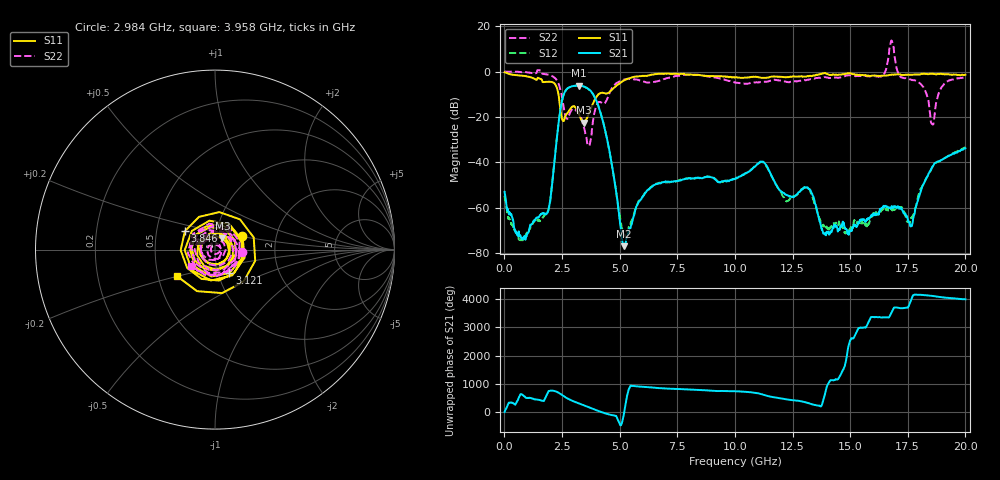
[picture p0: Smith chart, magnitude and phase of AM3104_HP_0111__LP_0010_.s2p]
!Created with skrf (http://scikit-rf.org).
# Hz S RI R 50.0
!freq ReS11 ImS11 ReS21 ImS21 ReS12 ImS12 ReS22 ImS22
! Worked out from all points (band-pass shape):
!   1601 points, 10 MHz to 20 GHz, reference 50 ohm
!   highest |S21| = -6.17 dB at 3.246 GHz (marker M1); lowest = -76.9 dB at 5.182 GHz (marker M2)
!   |S21| within 3 dB of the highest: 2.615 GHz to 3.791 GHz (1.177 GHz wide, 36.7 % of centre)
!   lowest |S11| = -22.5 dB at 3.458 GHz (marker M3), VSWR 1.16, Z = 53.9 + j6.82 ohm
!   |S11| at or under -10 dB: 2.347 GHz to 4.082 GHz (1.736 GHz wide, 54 % of centre)
!   |S22| runs from -32.7 to 13.7 dB; largest |S21 - S12| = 0.027
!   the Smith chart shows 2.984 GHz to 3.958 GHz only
!   S11 on the Smith chart (normalised r, x): 2.984 GHz: 1.34, +0.21; 3.121 GHz: 1.13, -0.30; 3.846 GHz: 0.70, +0.15; 3.958 GHz: 0.62, -0.20
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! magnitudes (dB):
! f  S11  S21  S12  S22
! 10 MHz  -0.3  -53.0  -54.7  0.0
! 722.1 MHz  -1.8  -73.1  -74.3  -0.2
! 1.834 GHz  -4.5  -62.5  -63.0  -1.2
! 2.496 GHz  -20.5  -13.0  -13.1  -11.1
! 2.984 GHz  -15.4  -6.3  -6.4  -16.5
! 3.121 GHz  -16.3  -6.2  -6.1  -17.4
! 3.246 GHz  -19.0  -6.2  -6.3  -18.8
! 3.346 GHz  -21.5  -6.3  -6.4  -20.6
! 3.458 GHz  -22.5  -6.6  -6.7  -24.9
! 3.846 GHz  -14.1  -9.9  -10.0  -21.6
! 3.958 GHz  -11.7  -12.1  -12.2  -15.9
! 5.182 GHz  -3.9  -76.9  -72.0  -3.6
! 6.682 GHz  -1.0  -49.3  -49.2  -4.2
! 10.01 GHz  -2.6  -47.3  -47.3  -4.8
! 11.18 GHz  -2.8  -39.7  -39.8  -4.6
! 12.22 GHz  -2.5  -54.3  -57.0  -4.5
! 13.34 GHz  -2.0  -53.7  -54.4  -3.3
! 13.92 GHz  -0.6  -71.8  -69.2  -2.5
! 16.68 GHz  -1.6  -60.1  -61.3  7.2
! 17.64 GHz  -1.4  -68.2  -64.6  -3.6
! 18.56 GHz  -0.9  -42.0  -42.0  -23.2
! 20 GHz  -1.4  -33.8  -33.4  -2.5
